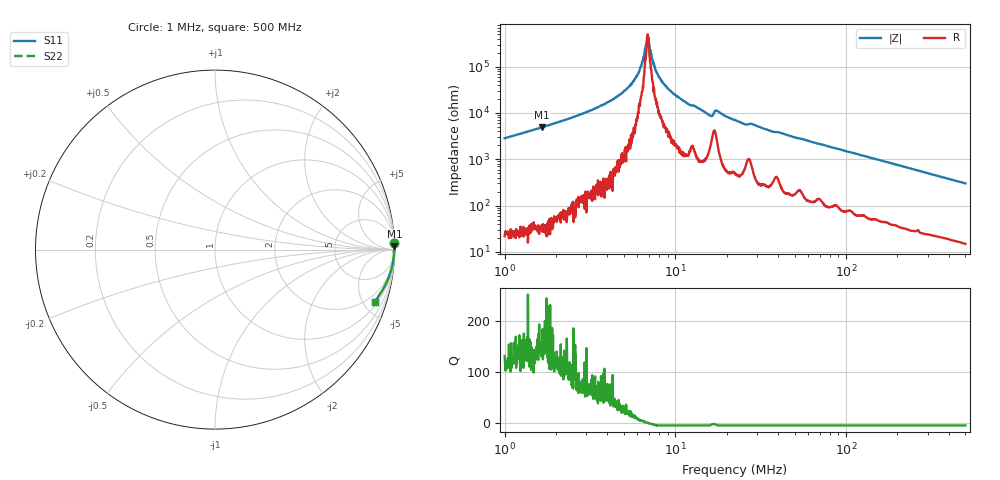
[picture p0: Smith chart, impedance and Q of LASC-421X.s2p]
!s-Parameter Generated by FASTRON Sdn. Bhd.
!FASTRON P/N : LASC-421X
!Keysight Technologies,E4991B,MY54100416,A.01.15
!Date: Tue Mar 17 15:59:58 2026
!Version  : Rev00 Tue Mar 17 15:59:58 2026
!Data & Calibration Information:
!PortZ  Port1:50+j0  Port2:50+j0
!When reading, reference impedance value at option line is always used.
!Remarks : This data is being provided solely for informational purposes.
!Freq	S11	S21	S12	S22
# Hz S dB R 50
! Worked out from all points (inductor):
!   1601 points, 1 MHz to 500 MHz, reference 50 ohm
!   read as one part in series: L = 444 uH near 1.032 MHz
!   highest Q = 157 at 1.657 MHz (marker M1), where L = 471 uH
!   self-resonance near 6.866 MHz
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1000000  -0.01 2.0  -29.08 -87.5  -29.08 -87.5  -0.01 2.0
1656881  -0.00 1.2  -33.81 -88.4  -33.81 -88.4  -0.00 1.2
2820919  -0.00 0.6  -39.53 -88.7  -39.53 -88.7  -0.00 0.6
4291124  -0.00 0.3  -45.76 -89.1  -45.76 -89.1  -0.00 0.3
5417295  -0.00 0.1  -51.85 -87.1  -51.85 -87.1  -0.00 0.1
6134256  -0.00 0.1  -58.04 -79.0  -58.04 -79.0  -0.00 0.1
6402024  -0.00 0.0  -61.72 -76.0  -61.72 -76.0  -0.00 0.0
6707483  -0.00 0.0  -68.77 -58.4  -68.77 -58.4  -0.00 0.0
6839020  -0.00 0.0  -72.83 -24.0  -72.83 -24.0  -0.00 0.0
7027516  -0.00 -0.0  -69.99 35.2  -69.99 35.2  -0.00 -0.0
7420238  -0.00 -0.0  -62.22 72.3  -62.22 72.3  -0.00 -0.0
7957584  -0.00 -0.1  -55.92 80.7  -55.92 80.7  -0.00 -0.1
9223203  -0.00 -0.2  -49.95 84.3  -49.95 84.3  -0.00 -0.2
1.196468e7  -0.00 -0.4  -43.78 85.0  -43.78 85.0  -0.00 -0.4
1.594882e7  -0.02 -0.6  -38.89 78.0  -38.89 78.0  -0.02 -0.6
1.757519e7  -0.02 -0.5  -40.91 77.3  -40.91 77.3  -0.02 -0.5
2.236068e7  -0.01 -0.8  -36.96 85.2  -36.96 85.2  -0.01 -0.8
2.55175e7  -0.02 -1.0  -35.14 82.8  -35.14 82.8  -0.02 -1.0
2.822906e7  -0.02 -1.0  -35.23 82.8  -35.23 82.8  -0.02 -1.0
6.307767e7  -0.03 -2.4  -27.50 84.7  -27.50 84.7  -0.03 -2.4
1.77937e8  -0.11 -6.7  -18.69 80.5  -18.69 80.5  -0.11 -6.7
5e8  -0.58 -18.0  -10.17 69.1  -10.17 69.1  -0.58 -18.0
